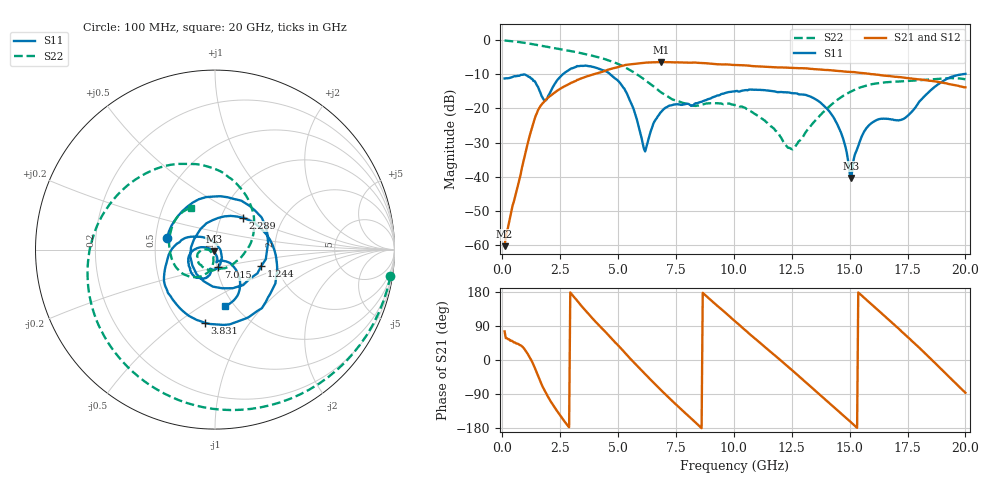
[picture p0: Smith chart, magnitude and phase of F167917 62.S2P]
!  2-Port S-parameters saved by WinCal
! VAR MeasName=S-Parameters (CALIBRATED_DATA) read from VNA (N5242A)
! VAR MeasDate=2016-11-22 9:03:06
! VAR NAME=F167917 62
! VAR FILENAME=F167917 62.S2P
! VAR DATE=2016-11-22 9:03:06
! VAR PHYS_PORTS=1,2
# Hz S DB R 50
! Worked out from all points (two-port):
!   401 points, 100 MHz to 20 GHz, reference 50 ohm
!   highest |S21| = -6.42 dB at 6.866 GHz (marker M1); lowest = -60.3 dB at 100 MHz (marker M2)
!   |S21| within 3 dB of the highest: 4.251 GHz to 15.24 GHz (10.99 GHz wide, 113 % of centre)
!   lowest |S11| = -40.4 dB at 15.07 GHz (marker M3), VSWR 1.02, Z = 49.6 - j0.845 ohm
!   |S11| at or under -10 dB: start of sweep to 2.614 GHz; 4.656 GHz to 19.88 GHz (15.22 GHz wide, 124 % of centre)
!   |S22| runs from -32.0 to -0.1 dB; largest |S21 - S12| = 0.0047
!   S11 on the Smith chart (normalised r, x): 100 MHz: 0.58, +0.08; 1.244 GHz: 1.65, -0.33; 2.289 GHz: 1.27, +0.48; 3.831 GHz: 0.65, -0.64; 7.015 GHz: 1.02, -0.20; 20 GHz: 0.91, -0.64
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1e8  -11.23 165.9  -60.34 75.3  -60.55 80.8  -0.10 -8.7
6.97e8  -10.46 76.4  -41.98 42.1  -41.99 41.8  -0.53 -55.9
1.24425e9  -11.26 -19.6  -26.57 0.4  -26.59 0.8  -1.10 -94.1
1.74175e9  -16.90 -164.7  -18.48 -70.3  -18.45 -70.1  -1.71 -123.8
2.289e9  -12.56 48.8  -15.22 -127.7  -15.22 -127.6  -2.36 -151.9
3.43325e9  -7.54 -67.9  -11.16 141.6  -11.11 141.9  -3.87 157.5
3.83125e9  -7.69 -97.6  -10.24 114.0  -10.17 114.1  -4.48 141.1
5.22425e9  -13.89 168.4  -7.47 23.9  -7.44 23.6  -7.74 79.3
6.11975e9  -31.86 50.0  -6.63 -33.9  -6.63 -34.1  -11.47 35.0
6.7665e9  -21.89 -67.5  -6.43 -73.9  -6.44 -73.9  -14.83 1.5
6.866e9  -20.98 -72.7  -6.42 -79.9  -6.43 -80.0  -15.34 -3.4
7.01525e9  -19.96 -79.7  -6.44 -89.0  -6.45 -89.0  -15.95 -10.5
8.458e9  -18.36 -100.2  -6.65 -171.6  -6.63 -171.6  -19.19 -84.5
1.005e10  -14.99 -116.3  -7.27 102.4  -7.25 102.4  -19.00 -149.8
1.2438e10  -15.43 -150.0  -8.15 -22.9  -8.12 -23.2  -31.67 -147.9
1.338325e10  -16.80 -168.7  -8.42 -74.1  -8.41 -74.1  -24.59 -98.6
1.437825e10  -23.49 168.1  -8.96 -127.6  -8.95 -127.6  -17.94 -105.7
1.507475e10  -40.36 -117.3  -9.32 -165.0  -9.33 -165.2  -15.01 -121.2
1.57215e10  -25.82 -75.3  -9.76 159.2  -9.78 159.3  -13.32 -138.5
1.67165e10  -23.15 -82.5  -10.49 104.9  -10.53 105.1  -12.27 -163.3
1.835825e10  -15.59 -44.2  -11.79 11.6  -11.71 11.8  -11.59 163.3
2e10  -9.89 -79.9  -13.82 -86.5  -13.68 -86.4  -11.47 120.6
